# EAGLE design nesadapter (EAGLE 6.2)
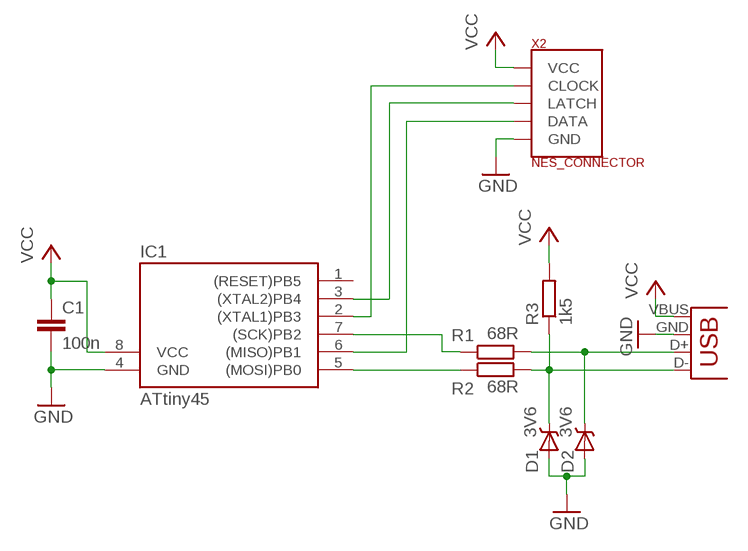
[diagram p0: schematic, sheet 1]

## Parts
C1  100n  C-EU050-024X044  [C050-024X044]
D1  3V6  DIODE_ZENER-DO35-6  [DO35-6]
D2  3V6  DIODE_ZENER-DO35-6  [DO35-6]
IC1  ATtiny45  TINY12P  [DIL08]
R1  68R  R-EU_0207/7  [0207/7]
R2  68R  R-EU_0207/7  [0207/7]
R3  1k5  R-EU_0207/7  [0207/7]
X1  USB-A-H  [USB-A-H]
X2  NES_CONNECTOR  [NES_CONNECTOR_EDGE]

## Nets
GND: C1.2 D1.A D2.A IC1.4(GND) X1.GND(VBUS) X2.P$1(GND)
N$1: D2.C R1.2 X1.D+(D-)
N$2: D1.C R2.2 R3.1 X1.D-(D+)
N$3: IC1.2((XTAL1)PB3) X2.P$2(CLOCK)
N$4: IC1.3((XTAL2)PB4) X2.P$3(LATCH)
N$5: IC1.6((MISO)PB1) X2.P$4(DATA)
N$6: IC1.7((SCK)PB2) R1.1
N$7: IC1.5((MOSI)PB0) R2.1
VCC: C1.1 IC1.8(VCC) R3.2 X1.VBUS(GND) X2.P$7(VCC)
Unconnected: IC1.1((RESET)PB5)

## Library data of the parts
C1 = rcl:C-EU: CAPACITOR, European symbol
D1 D2 = Bidouille:DIODE_ZENER: DIODE ZENER
IC1 = atmel:TINY12*: MICROCONTROLLER 1 Kbytes FLASH 64 bytes EEPROM; OC_FARNELL: unknown; OC_NEWARK: unknown
R1-R3 = rcl:R-EU_: RESISTOR, European symbol
X1 = SparkFun:USB: USB Connectors USB-B-PTH is fully proven SKU : PRT-00139 USB-miniB is fully proven SKU : PRT-00587 USB-A-PCB is untested. USB-A-H is throughly reviewed, but untested. Spark Fun Electronics SKU : PRT-00437 USB-B-SMT is throughly reviewed, but untested. Needs silkscreen touching up. USB-A-S has not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
X2 = Bidouille:NES_CONNECTOR

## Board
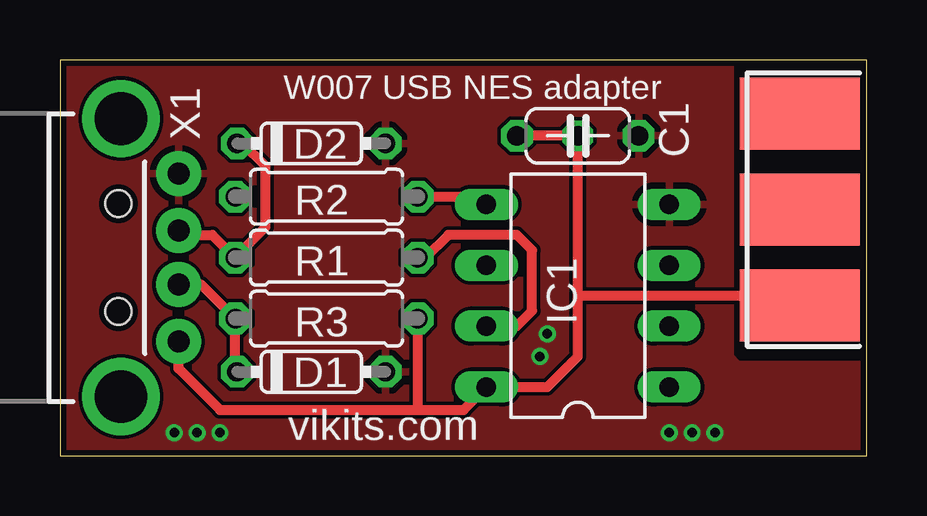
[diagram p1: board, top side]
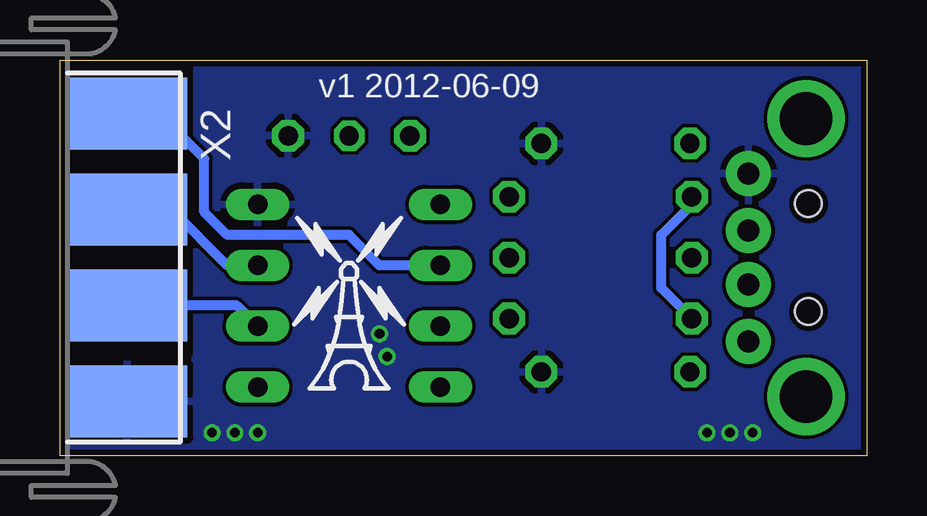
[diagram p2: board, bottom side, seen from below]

Size 33.64 x 16.5 mm. Coordinates in mm from the lower left corner, seen from the top.
Outline: 0,0 33.64,0 33.64,16.5 0,16.5 0,0
Copper layers (1*16): Top 0.035mm / dielectric 1.5mm / Bottom 0.035mm
Design rules: minimum track width 6mil, minimum drill 12mil, track to track 6mil, track to pad 6mil, pad to pad 6mil, via to via 6mil, smd to smd 0mil, copper to edge 10mil, drill to drill 10mil, minimum pad ring 10mil, minimum via ring 6mil, stop-mask expansion 2mil, vias tented up to drill 100mil, thermal gap 10mil

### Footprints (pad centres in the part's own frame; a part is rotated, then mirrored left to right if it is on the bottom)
C050-024X044 = drill 0.813 octagon: 1 -2.54,0; 2 2.54,0
DO35-6 = drill 0.8 octagon: A 3.1,0; C -3.1,0
DIL08 = drill 0.813 long: 1 -3.81,-3.81; 2 -1.27,-3.81; 3 1.27,-3.81; 4 3.81,-3.81; 5 3.81,3.81; 6 1.27,3.81; 7 -1.27,3.81; 8 -3.81,3.81
0207/7 = drill 0.813 octagon: 1 -3.81,0; 2 3.81,0
USB-A-H = drill 0.914 pad 1.88: D+ 2.4,1.127; D- 2.4,-1.127; GND 2.4,3.5; VBUS 2.4,-3.5 | drill 2.2: GND2 0,-5.8; GND3 0,5.8 | hole 1.1: -0.1,2.25; -0.1,-2.25
NES_CONNECTOR_EDGE = smd 5 x 3: P$1 -2.5,6; P$2 -2.5,2; P$3 -2.5,-2; P$4 -2.5,-6 | smd 5 x 3 bottom: P$5 -2.5,-6; P$6 -2.5,-2; P$7 -2.5,2

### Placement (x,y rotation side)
C1  21.59,13.34 0 top
D1  10.48,3.49 0 top
D2  10.48,13.02 0 top
IC1  21.59,6.67 90 top
R1  11.11,8.26 180 top
R2  11.11,10.79 180 top
R3  11.11,5.71 0 top
U$1  [LOGO_TOWER]  21.59,6.35 0 bottom
X1  2.54,8.26 0 top
X2  33.34,8.26 180 bottom

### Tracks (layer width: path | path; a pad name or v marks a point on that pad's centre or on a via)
GND  (via drill 0.4)
  other vias: 27.3,0.95 26.35,0.95 25.4,0.95 4.76,0.95 5.71,0.95 6.67,0.95 20.32,5.08 20,4.13
  pour Bottom: 0,0 0,16.51 27.94,16.51 27.94,4.13 28.26,3.81 33.34,3.81 33.34,0
  pour Top: 0,0 0,16.51 27.94,16.51 27.94,4.13 28.26,3.81 33.34,3.81 33.34,0
N$1
  Top 0.406: D2.C 7.62,13.02 8.57,12.06 8.57,9.53 R1.2 6.35,9.21 5.11,9.21 X1.D+
N$2
  Top 0.406: X1.D- 5.89,7.13 R3.1 7.3,3.57 D1.C
  Bottom 0.406: R2.2 7.3,10.48 8.57,9.21 8.57,6.99 R3.1
N$3
  Bottom 0.406: X2.P$2 26.26,6.25 IC1.2
N$4
  Bottom 0.406: X2.P$3 28.99,10.26 26.67,7.94 IC1.3
N$5
  Bottom 0.406: X2.P$4 29.49,14.26 27.62,12.38 27.62,10.16 26.67,9.21 21.59,9.21 20.32,7.94 IC1.6
N$6
  Top 0.406: R1.1 15.24,8.26 16.19,9.21 19.05,9.21 19.69,8.57 19.69,6.03 19.05,5.4 IC1.7
N$7
  Top 0.406: R2.1 17.46,10.79 IC1.5
VCC  (via drill 0.8 pad 1.27)
  Top 0.406: 21.59,6.67 v21.59,13.34 C1.1 | 21.59,6.67 21.59,4.13 20.32,2.86 IC1.8 16.83,1.91 14.92,1.91 | X2.P$7 30.26,6.25 29.85,6.67 21.59,6.67 | X1.VBUS 4.94,3.63 6.67,1.91 14.92,1.91 | 14.92,1.91 R3.2

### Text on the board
tNames: W007 USB NES adapter | vikits.com
bNames: v1 2012-06-09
